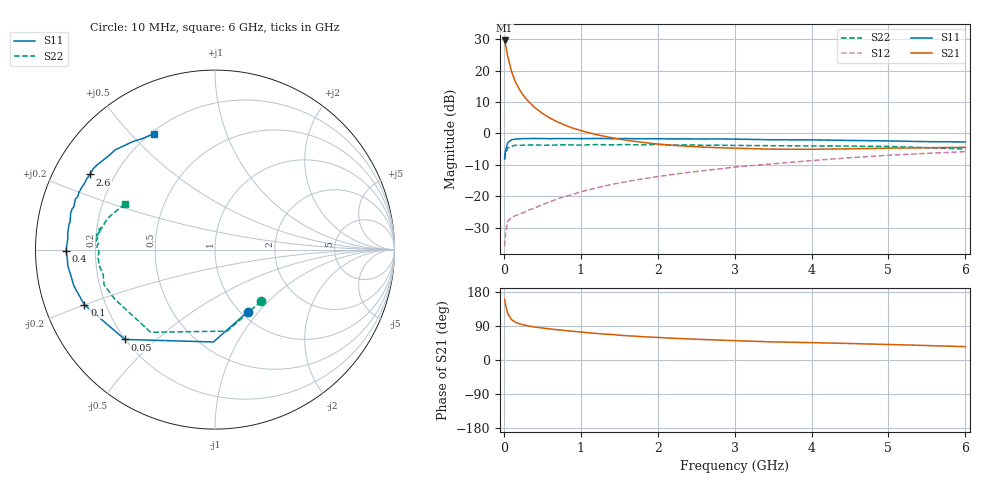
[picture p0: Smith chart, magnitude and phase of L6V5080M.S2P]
!  INFINEON TECHNOLOGIES Small Signal Semiconductors
! BFR380L3 , Si-NPN RF-Transistor in TSLP-3-1
!  Vce=0.5 V,  Ic=80 mA
! Common Emitter S-Parameters:  07. March 2005
#  GHz  S  MA  R  50
! f  S11  S21  S12  S22
! GHz  Mag  Ang  Mag  Ang  Mag  Ang  Mag  Ang
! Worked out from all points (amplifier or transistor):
!   36 points, 10 MHz to 6 GHz, reference 50 ohm
!   highest |S21| = 29.6 dB at 10 MHz (marker M1)
!   |S21| within 3 dB of that: start of sweep to 34.73 MHz
!   unconditionally stable (mu >= 1): 466.1 MHz to end of sweep
!   at 250 MHz: K = 0.73, MSG = 18.8 dB, |S12| = -25.3 dB
!   at 1.4 GHz: K = 1.23, MAG = 4.5 dB, |S12| = -16.3 dB
!   at 6 GHz: K = 1.07, MAG = -1.0 dB, |S12| = -5.8 dB
!   S11 on the Smith chart (normalised r, x): 10 MHz: 1.07, -0.88; 50 MHz: 0.20, -0.40; 100 MHz: 0.12, -0.20; 400 MHz: 0.09, -0.00; 2.6 GHz: 0.11, +0.27; 6 GHz: 0.21, +0.58
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0.01  0.3915 -62.2  30.09 160.3  0.016 47.2  0.3856 -48.4
0.02  0.5147 -91.0  26.55 148.3  0.0245 45.6  0.4593 -81.5
0.05  0.7091 -135.1  16.95 122.6  0.0398 33.7  0.5838 -127.9
0.1  0.7902 -157.1  9.647 106.5  0.0455 28.0  0.624 -154.0
0.15  0.812 -165.6  6.617 99.6  0.049 28.4  0.6484 -162.4
0.2  0.8166 -170.1  5.042 95.8  0.0517 31.8  0.6384 -167.2
0.25  0.8253 -173.7  4.081 92.8  0.0543 33.9  0.6479 -171.2
0.3  0.8239 -175.6  3.409 90.7  0.0585 37.4  0.6499 -172.5
0.4  0.8295 -179.6  2.582 87.1  0.065 42.4  0.6549 -176.4
0.5  0.8252 177.8  2.086 84.4  0.0733 46.8  0.6474 -178.1
0.6  0.822 175.8  1.741 82.0  0.0815 50.1  0.6477 -179.1
0.7  0.8252 174.2  1.517 79.7  0.0907 53.1  0.6527 179.5
0.9  0.8258 170.3  1.206 75.8  0.107 56.4  0.6542 177.4
1.1  0.8253 167.6  1.026 71.9  0.1264 58.4  0.6579 176.7
1.3  0.8276 164.1  0.902 68.3  0.1446 59.0  0.6587 174.2
1.6  0.8272 160.1  0.774 64.0  0.171 59.7  0.6638 172.8
2.2  0.8157 153.1  0.645 57.3  0.222 59.6  0.649 171.4
2.6  0.8128 149.0  0.603 54.0  0.2549 59.1  0.645 170.5
3.5  0.7896 138.5  0.56 47.8  0.3281 55.5  0.6355 167.5
4.5  0.7712 131.7  0.567 43.6  0.4089 51.3  0.6267 164.6
5.5  0.7377 122.7  0.59 38.2  0.4802 45.0  0.5912 158.7
6  0.7293 117.8  0.599 35.2  0.5115 42.1  0.5617 152.8
